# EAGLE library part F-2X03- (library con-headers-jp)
FEMALE HEADER
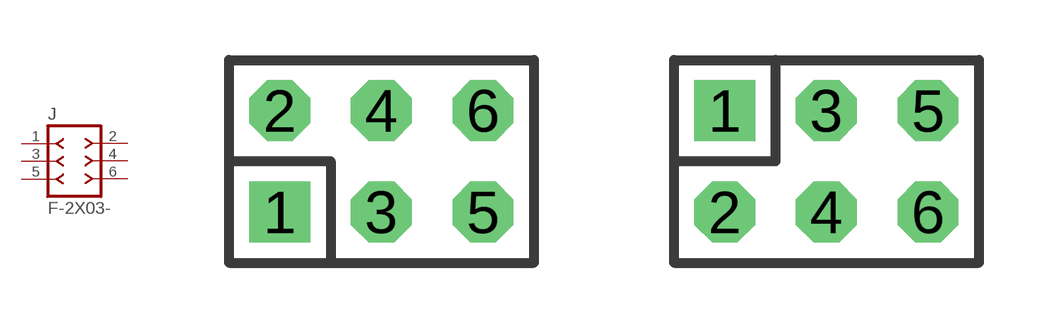
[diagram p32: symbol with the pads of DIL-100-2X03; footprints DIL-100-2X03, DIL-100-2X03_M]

Designator prefix J

## F-2X03-DIL-100  [DIL-100-2X03]
1  1  pas
2  2  pas
3  3  pas
4  4  pas
5  5  pas
6  6  pas

## F-2X03-DIL-100_M  [DIL-100-2X03_M]
Pads as for DIL-100-2X03

## F-2X03-DIL-2MM  [DIL-2MM-2X03]
Pads as for DIL-100-2X03

## F-2X03-DIL-2MM_M  [DIL-2MM-2X03_M]
Pads as for DIL-100-2X03

## F-2X03-79107  [79107-06]
Pads as for DIL-100-2X03

## F-2X03-79107_M  [79107-06_M]
Pads as for DIL-100-2X03

## Footprint DIL-100-2X03 (pad centres in mm)
PIN HEADER - 0.1"
drill 1.016 square: 1 -2.54,-1.27
drill 1.016 octagon: 2 -2.54,1.27; 3 0,-1.27; 4 0,1.27; 5 2.54,-1.27; 6 2.54,1.27

## Footprint DIL-100-2X03_M (pad centres in mm)
PIN HEADER - MIRRORED 0.1"
drill 1.016 square: 1 -2.54,1.27
drill 1.016 octagon: 2 -2.54,-1.27; 3 0,1.27; 4 0,-1.27; 5 2.54,1.27; 6 2.54,-1.27

## Footprint DIL-2MM-2X03 (pad centres in mm)
PIN HEADER - 2MM"
drill 0.711 square: 1 -2,-1
drill 0.711: 2 -2,1; 3 0,-1; 4 0,1; 5 2,-1; 6 2,1

## Footprint DIL-2MM-2X03_M (pad centres in mm)
PIN HEADER - MIRRORED 2MM
drill 0.711 square: 1 -2,1
drill 0.711: 2 -2,-1; 3 0,1; 4 0,-1; 5 2,1; 6 2,-1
